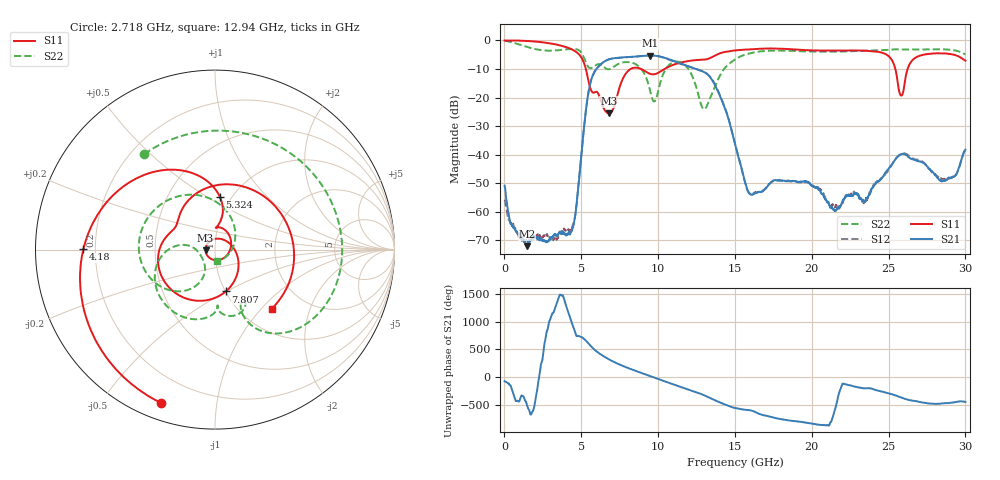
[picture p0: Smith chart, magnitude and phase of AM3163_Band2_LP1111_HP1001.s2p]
!Agilent Technologies,E8364B,MY43040894,A.07.50.67
!Agilent E8364B: A.07.50.67
!Date: Thursday, August 20, 2020 12:09:08
!Correction: S11(Full 2 Port(1,2))
!S21(Full 2 Port(1,2))
!S12(Full 2 Port(1,2))
!S22(Full 2 Port(1,2))
!S2P File: Measurements: S11, S21, S12, S22:
# Hz S  dB  R 50
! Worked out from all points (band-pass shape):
!   3201 points, 10 MHz to 30 GHz, reference 50 ohm
!   highest |S21| = -5.31 dB at 9.504 GHz (marker M1); lowest = -72.0 dB at 1.472 GHz (marker M2)
!   |S21| within 3 dB of the highest: 6.281 GHz to 11.57 GHz (5.294 GHz wide, 59.3 % of centre)
!   lowest |S11| = -25.5 dB at 6.786 GHz (marker M3), VSWR 1.11, Z = 45 - j0.277 ohm
!   |S11| at or under -10 dB: 5.296 GHz to 8.217 GHz (2.921 GHz wide, 43.2 % of centre); 8.88 GHz to 10.43 GHz (1.55 GHz wide, 16.1 % of centre); 25.44 GHz to 26.24 GHz (800.6 MHz wide, 3.1 % of centre)
!   |S22| runs from -24.1 to -0.2 dB; largest |S21 - S12| = 0.013
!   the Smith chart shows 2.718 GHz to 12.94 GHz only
!   S11 on the Smith chart (normalised r, x): 2.718 GHz: 0.07, -0.71; 4.18 GHz: 0.15, +0.00; 5.324 GHz: 0.88, +0.57; 7.807 GHz: 1.00, -0.50; 12.94 GHz: 1.38, -1.15
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1e7  -0.05 -2.6  -50.87 -75.2  -55.71 25.5  -0.16 -6.9
1.472012e9  -0.21 -58.0  -72.01 -154.9  -70.42 130.9  -2.31 -134.9
2.718472e9  -0.86 -109.3  -70.59 58.4  -67.99 -157.9  -3.58 126.6
4.180484e9  -2.69 179.9  -67.14 74.3  -66.54 -86.7  -3.08 19.8
5.014581e9  -6.06 116.6  -39.54 2.6  -39.58 2.0  -4.38 -50.0
5.323853e9  -10.60 84.7  -23.44 -67.6  -23.50 -68.0  -8.02 -66.8
6.148578e9  -19.14 42.3  -8.99 72.8  -9.05 72.6  -8.33 -73.2
6.785866e9  -25.51 -176.7  -6.67 -37.8  -6.70 -37.9  -10.13 -87.3
7.8074e9  -12.38 -75.5  -5.92 -170.1  -5.98 -169.9  -7.65 -115.2
9.503709e9  -11.77 154.7  -5.31 14.4  -5.30 14.3  -18.15 174.2
1.000979e10  -11.36 138.3  -5.55 -36.9  -5.57 -37.4  -17.64 -115.3
1.134997e10  -7.95 50.4  -7.86 -166.1  -8.07 -165.0  -7.49 163.5
1.294319e10  -6.79 -45.9  -10.97 36.8  -10.93 38.3  -23.99 -78.1
1.5005e10  -3.53 -132.3  -36.39 160.6  -36.31 160.3  -6.70 -112.2
1.596093e10  -3.20 -172.2  -53.70 121.1  -53.65 118.9  -4.58 -170.0
1.787279e10  -2.89 98.3  -48.97 -35.5  -48.98 -37.2  -3.58 92.1
2.000958e10  -3.51 -9.8  -50.99 -121.5  -50.35 -120.5  -3.94 -9.5
2.231506e10  -3.56 -100.1  -54.30 -138.4  -54.40 -128.6  -3.86 -93.8
2.500479e10  -5.54 158.0  -44.86 64.8  -45.32 65.1  -3.36 -167.6
2.582014e10  -19.33 170.6  -39.86 -9.8  -39.81 -7.0  -3.21 170.3
2.727278e10  -5.03 156.9  -42.95 -104.0  -42.75 -103.8  -3.19 133.1
3e10  -7.09 51.5  -38.23 -88.6  -38.16 -88.5  -4.89 55.1
